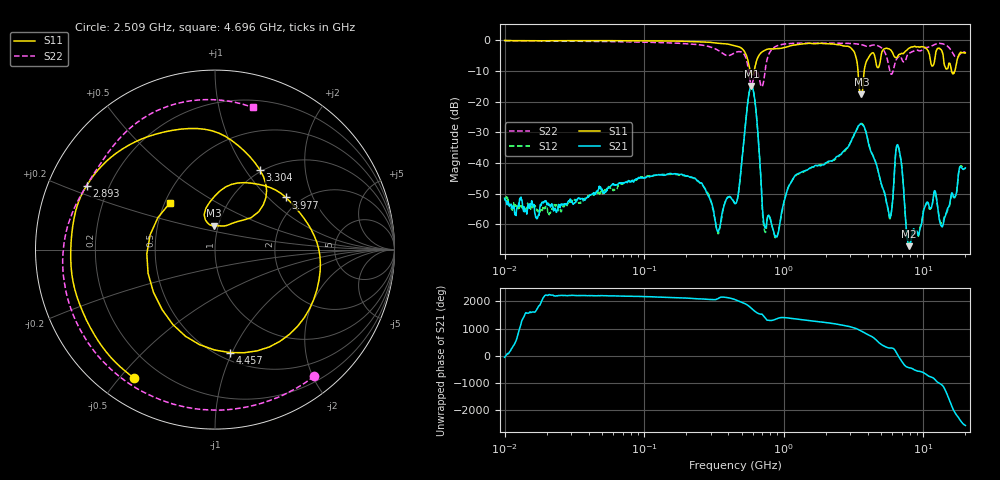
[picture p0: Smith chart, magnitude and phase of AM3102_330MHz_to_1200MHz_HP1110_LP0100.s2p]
! Date/Time: Tue, Sep 11, 2018 5:23 PM
! Network Analyzer: Agilent Technologies E8362B Rev: A.07.50.63
! Sweep from 0.010 to 20.000 GHz, 1601 Points, Sweep Type: LOG
! Power Supply: 4.949 V, 0.001 A
# Hz S DB R 50
!freq MagS11 AngS11 MagS21 AngS21 MagS12 AngS12 MagS22 AngS22
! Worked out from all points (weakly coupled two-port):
!   1601 points, 10 MHz to 20 GHz, reference 50 ohm
!   highest |S21| = -14.87 dB at 586.3 MHz (marker M1); lowest = -67.1 dB at 7.882 GHz (marker M2)
!   lowest |S11| = -17.5 dB at 3.599 GHz (marker M3), VSWR 1.31, Z = 47.8 + j12.9 ohm
!   |S11| at or under -10 dB: 574.8 MHz to 611.8 MHz (37 MHz wide, 6.24 % of centre); 3.402 GHz to 3.767 GHz (365.7 MHz wide, 10.2 % of centre); 15.92 GHz to 16.81 GHz (890.4 MHz wide, 5.44 % of centre)
!   |S22| runs from -15.1 to -0.2 dB; largest |S21 - S12| = 0.0052
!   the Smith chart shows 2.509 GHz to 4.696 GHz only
!   S11 on the Smith chart (normalised r, x): 2.509 GHz: 0.11, -0.55; 2.893 GHz: 0.12, +0.23; 3.304 GHz: 0.97, +1.17; 3.977 GHz: 1.69, +1.29; 4.457 GHz: 0.57, -0.98; 4.696 GHz: 0.53, +0.32
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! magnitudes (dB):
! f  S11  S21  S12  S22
! 10 MHz  0.0  -51.5  -51.8  -0.2
! 35.55 MHz  -0.1  -51.6  -52.9  -0.3
! 126.4 MHz  -0.2  -43.8  -43.9  -0.7
! 254.1 MHz  -0.5  -46.4  -46.8  -1.5
! 337.9 MHz  -1.0  -62.3  -63.0  -3.2
! 447.2 MHz  -1.8  -53.2  -53.2  -4.0
! 586.3 MHz  -11.2  -14.9  -15.0  -14.2
! 733 MHz  -3.2  -61.1  -62.4  -10.2
! 890.6 MHz  -2.7  -64.0  -64.3  -1.8
! 1.113 GHz  -1.8  -46.8  -46.6  -1.0
! 1.59 GHz  -1.0  -41.3  -41.3  -0.9
! 2.509 GHz  -1.5  -37.3  -37.6  -1.0
! 2.893 GHz  -1.9  -34.7  -34.5  -1.0
! 3.304 GHz  -5.8  -29.4  -29.4  -1.1
! 3.599 GHz  -17.5  -27.3  -27.1  -1.4
! 3.977 GHz  -6.2  -32.2  -32.0  -2.0
! 4.457 GHz  -4.7  -38.7  -38.6  -1.5
! 4.696 GHz  -8.8  -41.9  -41.9  -1.7
! 5.652 GHz  -2.7  -56.3  -56.7  -8.4
! 6.612 GHz  -4.8  -34.6  -34.6  -5.4
! 7.882 GHz  -2.6  -67.1  -66.3  -4.3
! 20 GHz  -4.1  -41.6  -41.9  -3.8
